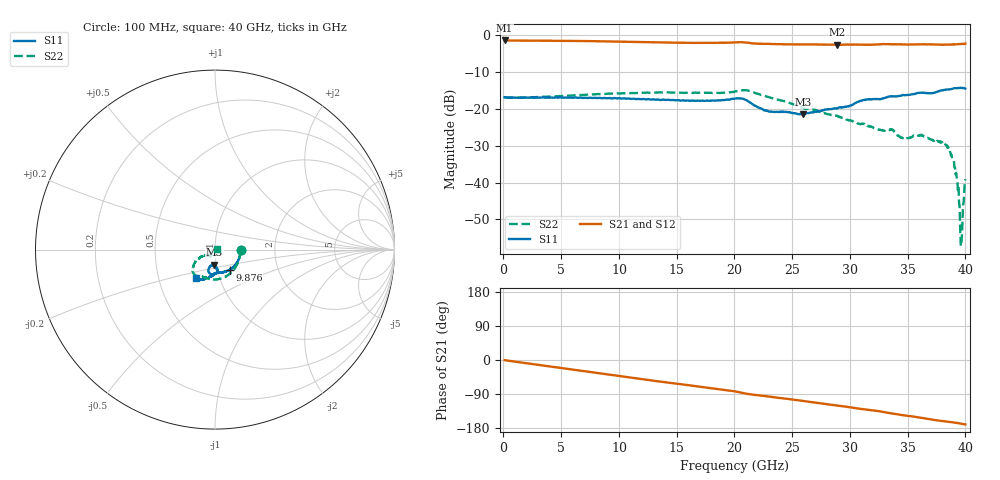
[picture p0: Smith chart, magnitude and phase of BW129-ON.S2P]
!  2-Port S-parameters saved by WinCal
! VAR MeasName=S-Parameters (CALIBRATED_DATA) read from VNA (N5244A)
! VAR MeasDate=5/25/2013 11:23:10 AM
! VAR NAME=132606
! VAR FILENAME=132606.S2P
! VAR DATE=5/25/2013 11:23:10 AM
! VAR PHYS_PORTS=1,2
# Hz S MA R 50
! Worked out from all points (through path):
!   801 points, 100 MHz to 40 GHz, reference 50 ohm
!   highest |S21| = -1.39 dB at 100 MHz (marker M1); lowest = -2.6 dB at 28.88 GHz (marker M2)
!   group delay of S21, straight-line fit = 11.7 ps
!   lowest |S11| = -21.5 dB at 25.94 GHz (marker M3), VSWR 1.18, Z = 48.8 - j8.29 ohm
!   |S11| at or under -10 dB: start of sweep to end of sweep
!   |S22| runs from -57.3 to -14.9 dB; largest |S21 - S12| = 0.02
!   S11 on the Smith chart (normalised r, x): 100 MHz: 1.34, -0.01; 9.876 GHz: 1.14, -0.27; 40 GHz: 0.77, -0.25
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1e8  0.1446 -1.0  0.8524 -0.5  0.8529 -0.5  0.1444 -1.2
6.78325e9  0.1421 -38.2  0.8373 -28.7  0.8379 -28.7  0.1552 -51.7
9.8755e9  0.1399 -54.5  0.8251 -41.7  0.827 -41.7  0.1625 -72.4
1.341662e10  0.1343 -69.8  0.804 -56.4  0.8076 -56.5  0.1676 -92.3
2.005e10  0.1385 -93.2  0.8045 -82.8  0.81 -82.6  0.1726 -120.9
2.10475e10  0.1318 -105.2  0.7967 -89.1  0.8081 -89.2  0.1797 -131.2
2.294275e10  0.0931 -104.8  0.7667 -96.2  0.7717 -96.7  0.1455 -144.4
2.593525e10  0.0844 -93.1  0.7565 -107.9  0.7595 -108.4  0.1033 -152.1
2.673325e10  0.08951 -89.6  0.7528 -111.5  0.7585 -111.8  0.09771 -150.8
2.887788e10  0.102 -86.7  0.7436 -120.1  0.7466 -120.8  0.08049 -152.1
3.231925e10  0.1359 -92.9  0.7522 -134.3  0.7553 -134.6  0.0535 -145.3
3.336662e10  0.1474 -95.0  0.7604 -139.9  0.7566 -140.2  0.05219 -138.0
3.46135e10  0.1544 -100.0  0.7544 -145.7  0.7547 -146.1  0.04019 -133.2
3.615962e10  0.1656 -106.4  0.7538 -152.4  0.7575 -153.0  0.04464 -125.1
3.8404e10  0.1847 -113.7  0.7481 -162.7  0.7532 -162.7  0.03213 -134.3
3.8803e10  0.1871 -115.9  0.7517 -163.9  0.7584 -164.5  0.02385 -142.7
3.910225e10  0.1919 -118.1  0.7572 -165.7  0.7655 -166.1  0.01598 -152.7
3.930175e10  0.193 -119.6  0.7578 -166.5  0.765 -167.3  0.01066 -158.3
3.950125e10  0.1926 -121.3  0.7601 -167.3  0.7666 -168.5  0.004759 -153.9
3.965088e10  0.1931 -122.7  0.7645 -168.3  0.7666 -169.3  0.001521 -122.2
3.975062e10  0.1936 -123.5  0.7633 -168.9  0.7667 -169.8  0.002983 -13.4
4e10  0.1892 -124.6  0.7688 -170.0  0.7629 -171.5  0.0111 3.6
